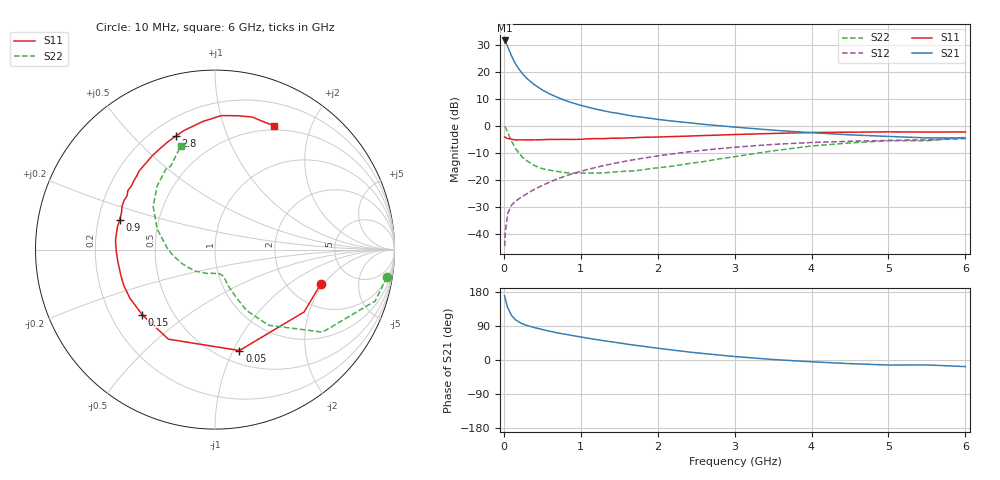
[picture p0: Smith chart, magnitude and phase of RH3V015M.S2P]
! SIEMENS Small Signal Semiconductors
! BFR106
! Si NPN RF Bipolar Junction Transistor in SOT23
! VCE = 3 V  IC = 15 mA
! Common Emitter S-Parameters:  August  1996
# GHz  S  MA  R  50
!  f  S11  S21  S12  S22
! GHz  MAG  ANG  MAG  ANG  MAG  ANG  MAG  ANG
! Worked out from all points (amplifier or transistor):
!   36 points, 10 MHz to 6 GHz, reference 50 ohm
!   highest |S21| = 31.5 dB at 10 MHz (marker M1)
!   |S21| within 3 dB of that: start of sweep to 59.97 MHz
!   unconditionally stable (mu >= 1): 405.4 MHz to 2.209 GHz; 5.201 GHz to end of sweep
!   at 250 MHz: K = 0.83, MSG = 22.5 dB, |S12| = -26.0 dB
!   at 1.4 GHz: K = 1.08, MAG = 7.9 dB, |S12| = -14.2 dB
!   at 6 GHz: K = 1.01, MAG = -0.4 dB, |S12| = -4.8 dB
!   S11 on the Smith chart (normalised r, x): 10 MHz: 2.99, -1.87; 50 MHz: 0.63, -1.06; 150 MHz: 0.33, -0.34; 900 MHz: 0.29, +0.14; 2.8 GHz: 0.29, +0.67; 6 GHz: 0.45, +1.48
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0.01  0.6196 -18.1  37.66 169.3  0.0059 84.6  0.9701 -9.0
0.02  0.6059 -35.0  36.07 160.4  0.011 75.1  0.9372 -17.8
0.05  0.5786 -76.4  28.84 137.9  0.0237 60.6  0.7554 -37.5
0.1  0.5626 -117.5  19.46 117.6  0.0339 50.8  0.5163 -54.7
0.15  0.5441 -138.2  14.04 106.3  0.0398 49.0  0.3815 -62.6
0.2  0.546 -150.2  10.93 99.8  0.0449 51.4  0.3054 -65.4
0.25  0.5463 -158.5  8.847 94.7  0.0499 52.9  0.2532 -67.8
0.3  0.544 -164.6  7.456 91.2  0.0552 55.2  0.2237 -69.4
0.4  0.5457 -173.3  5.676 85.4  0.0668 58.2  0.1824 -71.0
0.5  0.5504 -179.3  4.566 80.4  0.0783 60.4  0.1601 -72.0
0.6  0.5566 174.9  3.841 75.8  0.0911 62.1  0.1495 -74.1
0.7  0.5564 170.4  3.322 71.5  0.104 62.8  0.1418 -77.5
0.9  0.5564 162.6  2.616 64.2  0.1302 63.0  0.132 -83.1
1.1  0.5714 155.0  2.182 57.3  0.1561 62.3  0.1333 -92.1
1.3  0.5745 148.5  1.879 50.9  0.1828 60.7  0.1338 -100.7
1.6  0.5928 139.6  1.568 41.9  0.2223 57.9  0.1435 -115.7
2.2  0.6291 123.8  1.21 26.1  0.3015 50.3  0.1785 -145.9
2.8  0.6692 108.9  0.998 13.1  0.3752 41.4  0.2428 -174.5
3.5  0.7173 95.3  0.826 1.3  0.45 30.3  0.3422 160.4
4.5  0.757 80.2  0.676 -9.6  0.5138 14.5  0.4794 132.2
5.5  0.7616 68.5  0.594 -13.0  0.5461 4.2  0.5266 117.9
6  0.7646 64.7  0.593 -17.4  0.5748 -3.2  0.6078 108.3
